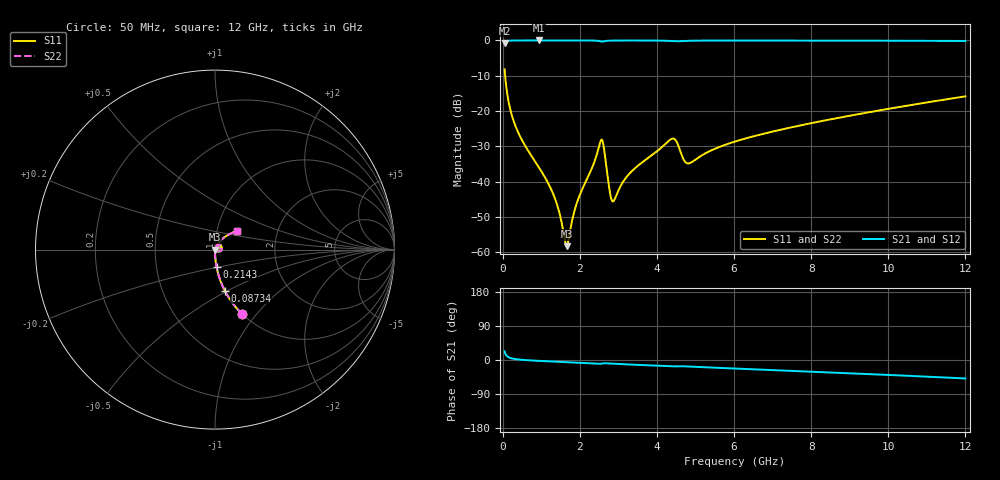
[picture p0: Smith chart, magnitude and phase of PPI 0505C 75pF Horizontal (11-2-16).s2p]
# MHz S MA R 50
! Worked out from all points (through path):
!   1601 points, 50 MHz to 12 GHz, reference 50 ohm
!   highest |S21| = -0.01 dB at 938.8 MHz (marker M1); lowest = -0.7 dB at 50 MHz (marker M2)
!   group delay of S21, straight-line fit = 11.6 ps
!   lowest |S11| = -58.3 dB at 1.656 GHz (marker M3), VSWR 1.00, Z = 50.1 - j0.0212 ohm
!   |S11| at or under -10 dB: 63.42 MHz to end of sweep
!   |S22| runs from -58.3 to -8.2 dB; largest |S21 - S12| = 0
!   S11 on the Smith chart (normalised r, x): 50 MHz: 1.00, -0.84; 87.34 MHz: 1.00, -0.48; 214.3 MHz: 1.00, -0.19; 12 GHz: 1.25, +0.27
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50  0.3893 -67.2  0.9208 22.7  0.9208 22.7  0.3893 -67.2
87.34375  0.2348 -76.6  0.9717 13.3  0.9717 13.3  0.2348 -76.6
214.3125  0.09674 -84.9  0.9948 4.8  0.9948 4.8  0.09674 -84.9
460.7812  0.04268 -88.3  0.9984 0.9  0.9984 0.9  0.04268 -88.3
938.7812  0.01593 -89.1  0.9989 -2.3  0.9989 -2.3  0.01593 -89.1
1357.031  0.005754 -83.7  0.9988 -4.3  0.9988 -4.3  0.005754 -83.7
1655.781  0.00122 -10.0  0.9987 -5.7  0.9987 -5.7  0.00122 -10.0
1879.844  0.004188 63.8  0.9985 -6.7  0.9985 -6.7  0.004188 63.8
2044.156  0.007405 69.6  0.9982 -7.4  0.9982 -7.4  0.007405 69.6
2552.031  0.03886 24.7  0.9676 -10.0  0.9676 -10.0  0.03886 24.7
2626.719  0.02964 -19.7  0.9707 -8.6  0.9707 -8.6  0.02964 -19.7
2791.031  0.00659 -16.7  0.9933 -9.5  0.9933 -9.5  0.00659 -16.7
2865.719  0.005258 18.9  0.9952 -9.9  0.9952 -9.9  0.005258 18.9
3283.969  0.01294 66.8  0.9972 -11.9  0.9972 -11.9  0.01294 66.8
4038.312  0.02796 64.6  0.9945 -15.3  0.9945 -15.3  0.02796 64.6
4434.156  0.04066 35.2  0.9742 -16.9  0.9742 -16.9  0.04066 35.2
4710.5  0.01978 22.9  0.9844 -16.7  0.9844 -16.7  0.01978 22.9
4830  0.01815 39.7  0.9897 -17.3  0.9897 -17.3  0.01815 39.7
6025  0.03697 62.7  0.9958 -22.5  0.9958 -22.5  0.03697 62.7
8019.156  0.06763 56.7  0.9942 -30.8  0.9942 -30.8  0.06763 56.7
10013.31  0.1077 48.8  0.9902 -39.4  0.9902 -39.4  0.1077 48.8
12000  0.1614 39.9  0.9822 -48.7  0.9822 -48.7  0.1614 39.9
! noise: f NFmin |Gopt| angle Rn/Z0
50  0.0003757  0.86  0.4473  0.0005749
1372  0.003877  0.6666  4.719  0.002227
2701  0.0187  0.8494  9.226  0.02627
4031  0.01394  0.7209  13.63  0.009757
5360  0.01483  0.6647  18.03  0.008276
6682  0.01417  0.5866  22.14  0.006045
8012  0.01571  0.564  26.2  0.006181
9341  0.01761  0.5546  30.15  0.006638
1.067e+04  0.0197  0.5518  33.98  0.007238
1.2e+04  0.02195  0.5537  37.68  0.007955
